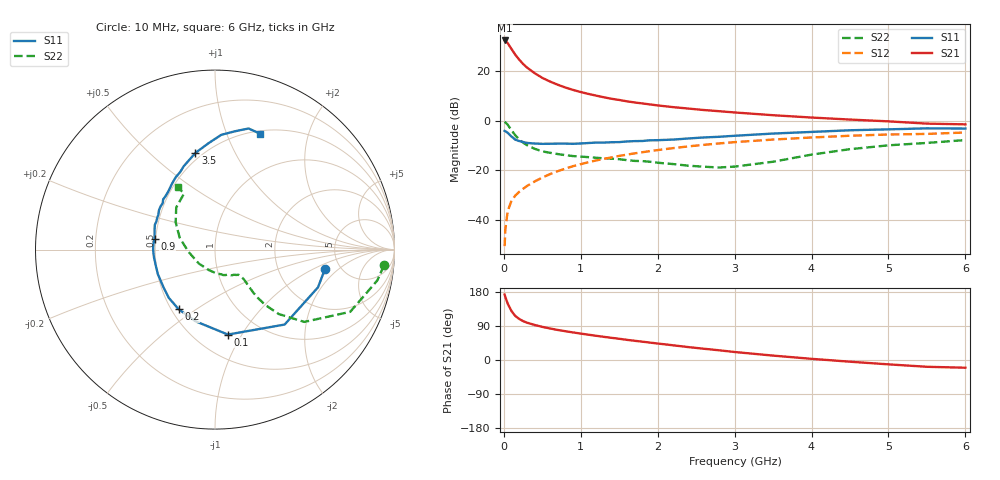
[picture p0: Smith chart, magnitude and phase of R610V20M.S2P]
! SIEMENS Small Signal Semiconductors
! BFR193
! Si NPN RF Bipolar Junction Transistor in SOT23
! VCE = 10 V  IC = 20 mA
! Common Emitter S-Parameters:  May  1996
# GHz  S  MA  R  50
!  f  S11  S21  S12  S22
! GHz  MAG  ANG  MAG  ANG  MAG  ANG  MAG  ANG
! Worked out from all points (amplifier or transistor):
!   36 points, 10 MHz to 6 GHz, reference 50 ohm
!   highest |S21| = 32.2 dB at 10 MHz (marker M1)
!   |S21| within 3 dB of that: start of sweep to 90.32 MHz
!   unconditionally stable (mu >= 1): 625.9 MHz to 2.205 GHz
!   at 250 MHz: K = 0.80, MSG = 25.1 dB, |S12| = -27.4 dB
!   at 1.4 GHz: K = 1.03, MAG = 10.7 dB, |S12| = -14.8 dB
!   at 6 GHz: K = 0.94, MSG = 1.6 dB, |S12| = -4.8 dB
!   S11 on the Smith chart (normalised r, x): 10 MHz: 3.81, -1.32; 100 MHz: 0.71, -0.87; 200 MHz: 0.55, -0.43; 900 MHz: 0.49, +0.07; 3.5 GHz: 0.46, +0.71; 6 GHz: 0.53, +1.32
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0.01  0.6227 -9.8  40.85 172.7  0.003 75.8  0.9453 -5.3
0.02  0.6112 -20.1  40.29 166.1  0.0066 78.0  0.921 -10.7
0.05  0.57 -47.1  36.11 148.9  0.0151 69.6  0.8294 -24.7
0.1  0.4787 -81.4  27.42 128.9  0.0248 62.2  0.6403 -39.0
0.15  0.4137 -105.3  21.02 116.0  0.0313 61.1  0.505 -45.3
0.2  0.3888 -121.5  16.79 108.3  0.0371 62.3  0.4183 -47.7
0.25  0.3723 -133.6  13.79 102.7  0.0426 62.6  0.3613 -48.4
0.3  0.3567 -143.0  11.72 98.5  0.0485 64.1  0.3223 -48.3
0.4  0.3465 -156.7  8.995 92.5  0.0599 66.0  0.2716 -47.3
0.5  0.3416 -165.5  7.238 87.4  0.0717 67.2  0.2414 -46.2
0.6  0.3428 -173.1  6.103 83.2  0.0841 67.5  0.2256 -45.8
0.7  0.3449 -179.5  5.272 79.3  0.0963 67.8  0.2131 -45.8
0.9  0.342 170.1  4.141 72.7  0.1215 66.9  0.1939 -46.7
1.1  0.3549 161.4  3.442 66.8  0.146 65.6  0.1845 -50.0
1.3  0.3623 154.5  2.948 61.1  0.1708 63.5  0.1748 -53.4
1.6  0.3818 144.8  2.444 53.2  0.2076 60.3  0.1607 -61.5
2.2  0.416 128.6  1.867 38.8  0.28 52.6  0.1341 -84.7
2.8  0.4736 114.2  1.546 25.6  0.3484 44.2  0.1144 -124.1
3.5  0.5499 101.4  1.285 11.6  0.4167 33.7  0.1493 -175.8
4.5  0.6402 86.9  1.051 -4.5  0.4971 19.8  0.267 145.2
5.5  0.7001 74.5  0.871 -17.9  0.5409 5.8  0.3563 119.0
6  0.6932 68.9  0.841 -20.4  0.5777 1.7  0.4074 120.6
